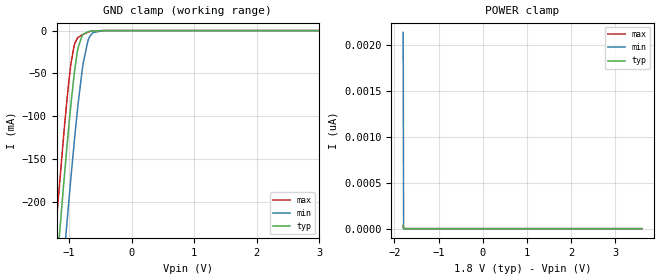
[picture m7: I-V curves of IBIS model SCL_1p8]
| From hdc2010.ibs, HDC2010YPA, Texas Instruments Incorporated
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[Model]   SCL_1p8
Model_type   Input
Vinl = 0.54
Vinh = 1.26
|   typ   min   max
|   (nom PVT)   (slow PVT)   (fast PVT)
C_comp   0.684p   0.665p   0.698p
[Model spec]
|subparameter
Vinl   0.54   0.486   0.594
Vinh   1.26   1.134   1.386
[Voltage Range]   1.8   1.62   1.98
[Temperature Range]   27   125   -40
[Power Clamp Reference]   1.8   1.62   1.98
[GND Clamp Reference]   0   0   0
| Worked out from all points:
|   GND clamp passes 1 mA (typ) near -0.68 V on its own axis
[GND Clamp]
|   Voltage   I(typ)   I(min)   I(max)
-1.8V     -845.7mA   -933.3mA   -789.9mA
-1.222V   -299.8mA   -390.8mA   -241.2mA
-1.184V   -265.8mA   -356.7mA   -207.2mA
-1.076V   -171.4mA   -261.4mA   -114.6mA
-1.033V   -135.6mA   -224.4mA   -80.85mA
-973.8mV  -89.32mA   -175.1mA   -41.29mA
-919.8mV  -52.42mA   -132.5mA   -18.11mA
-855mV    -20.02mA   -85.72mA   -8.028mA
-790.2mV  -5.792mA   -46.45mA   -5.02mA
-660.6mV  -779.7uA   -5.92mA    -1.007mA
-444.6mV  -4.708uA   -64.07uA   -1.274uA
3.6V      0A         0A         0A
[POWER Clamp]
|   Voltage   I(typ)   I(min)   I(max)
-1.8V     37.38pA    2.139nA    33.23pA
-1.789V   0A         0A         0A
-1.784V   0A         0A         0A
3.6V      0A         0A         0A
